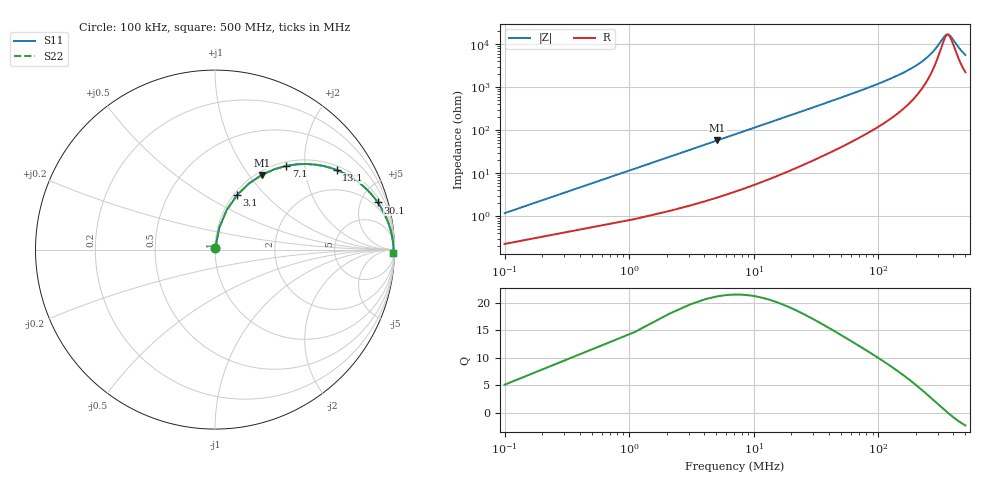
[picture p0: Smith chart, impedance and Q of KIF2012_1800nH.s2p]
!version-2
!date-12.2020
!Series
# MHz S RI R 50
!Freq ReS11 ImS11 ReS21 ImS21 ReS12 ImS12 ReS22 ImS22
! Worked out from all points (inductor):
!   501 points, 100 kHz to 500 MHz, reference 50 ohm
!   read as one part in series: L = 1.81 uH near 2.1 MHz
!   highest Q = 21.2 at 5.1 MHz (marker M1), where L = 1.8 uH
!   self-resonance near 361.2 MHz
!   S11 on the Smith chart (normalised r, x): 100 kHz: 1.00, +0.02; 3.1 MHz: 1.04, +0.70; 7.1 MHz: 1.07, +1.61; 13.1 MHz: 1.14, +2.95; 30.1 MHz: 1.40, +6.77; 500 MHz: open
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0.1  0.00242 0.0116  0.9976 -0.0116  0.9976 -0.0116  0.00242 0.0116
1.1  0.0238 0.1219  0.9762 -0.1219  0.9762 -0.1219  0.0238 0.1219
3.1  0.1227 0.3038  0.8773 -0.3038  0.8773 -0.3038  0.1227 0.3038
4.1  0.1897 0.3686  0.8103 -0.3686  0.8103 -0.3686  0.1897 0.3686
5.1  0.2605 0.4159  0.7395 -0.4159  0.7395 -0.4159  0.2605 0.4159
7.1  0.397 0.4666  0.603 -0.4666  0.603 -0.4666  0.397 0.4666
10.1  0.5624 0.4731  0.4376 -0.4731  0.4376 -0.4731  0.5624 0.4731
13.1  0.6777 0.4437  0.3223 -0.4437  0.3223 -0.4437  0.6777 0.4437
16.1  0.756 0.4051  0.244 -0.4051  0.244 -0.4051  0.756 0.4051
20.1  0.824 0.3554  0.176 -0.3554  0.176 -0.3554  0.824 0.3554
30.1  0.907 0.2625  0.093 -0.2625  0.093 -0.2625  0.907 0.2625
53.1  0.9626 0.157  0.0374 -0.157  0.0374 -0.157  0.9626 0.157
84.1  0.9811 0.0982  0.0189 -0.0982  0.0189 -0.0982  0.9811 0.0982
118.1  0.9879 0.0667  0.0121 -0.0667  0.0121 -0.0667  0.9879 0.0667
167.1  0.9917 0.0418  0.00828 -0.0418  0.00828 -0.0418  0.9917 0.0418
250.1  0.9938 0.0185  0.00619 -0.0185  0.00619 -0.0185  0.9938 0.0185
334.1  0.9941 0.00384  0.00588 -0.00384  0.00588 -0.00384  0.9941 0.00384
351.1  0.9941 0.00139  0.00592 -0.00139  0.00592 -0.00139  0.9941 0.00139
367.1  0.994 -0.000804  0.00599 0.000804  0.00599 0.000804  0.994 -0.000804
417.1  0.9937 -0.0071  0.00635 0.0071  0.00635 0.0071  0.9937 -0.0071
457.1  0.9932 -0.0117  0.00676 0.0117  0.00676 0.0117  0.9932 -0.0117
500  0.9927 -0.0162  0.00731 0.0162  0.00731 0.0162  0.9927 -0.0162
